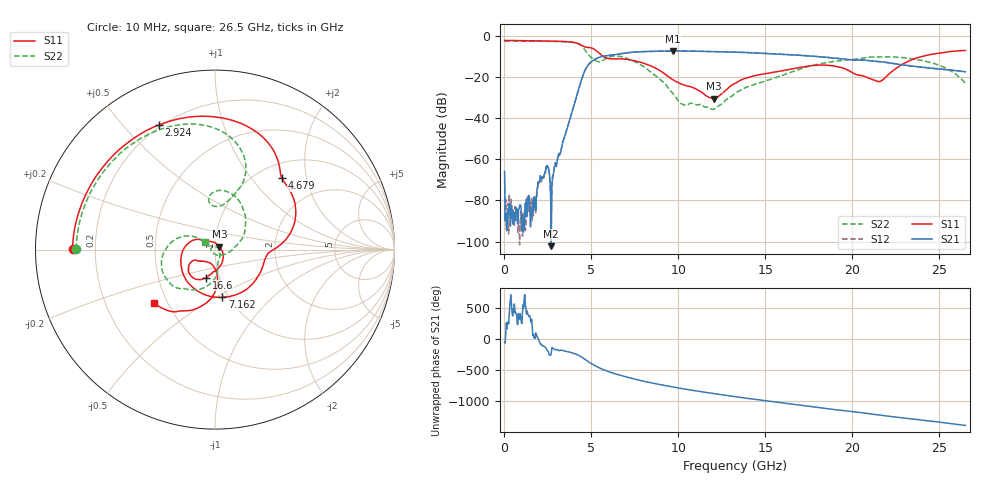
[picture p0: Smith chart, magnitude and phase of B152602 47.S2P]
!  2-Port S-parameters saved by WinCal
! VAR MeasName=S-Parameters (CALIBRATED_DATA) read from VNA (N5242A)
! VAR MeasDate=2016-1-5 16:32:53
! VAR NAME=B152602 47
! VAR FILENAME=B152602 47.S2P
! VAR DATE=2016-1-5 16:32:53
! VAR PHYS_PORTS=1,2
# Hz S DB R 50
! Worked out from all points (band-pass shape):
!   801 points, 10 MHz to 26.5 GHz, reference 50 ohm
!   highest |S21| = -7.09 dB at 9.679 GHz (marker M1); lowest = -102.3 dB at 2.692 GHz (marker M2)
!   |S21| within 3 dB of the highest: 5.494 GHz to 18.3 GHz (12.81 GHz wide, 108 % of centre)
!   lowest |S11| = -30.4 dB at 12.06 GHz (marker M3), VSWR 1.06, Z = 52.5 + j1.81 ohm
!   |S11| at or under -10 dB: 5.717 GHz to 23.92 GHz (18.2 GHz wide, 123 % of centre)
!   |S22| runs from -35.6 to -2.2 dB; largest |S21 - S12| = 0.0027
!   S11 on the Smith chart (normalised r, x): 10 MHz: 0.12, +0.00; 2.924 GHz: 0.19, +0.63; 4.679 GHz: 1.26, +1.44; 7.162 GHz: 0.93, -0.54; 16.6 GHz: 0.87, -0.28; 26.5 GHz: 0.42, -0.32
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1e7  -2.02 179.7  -65.84 -55.3  -70.16 -142.2  -2.24 179.8
1.755625e8  -2.02 176.4  -88.71 -84.1  -84.82 -162.3  -2.24 177.3
1.102712e9  -2.13 157.4  -94.88 143.0  -92.38 172.0  -2.30 162.9
1.73185e9  -2.20 143.9  -82.57 36.9  -82.17 30.6  -2.36 152.8
2.427212e9  -2.29 127.6  -64.22 -163.1  -64.13 -160.9  -2.44 140.5
2.692112e9  -2.32 120.7  -102.26 135.2  -88.88 -154.1  -2.46 135.4
2.9239e9  -2.36 114.2  -61.79 -168.0  -61.53 -163.7  -2.50 130.5
4.447075e9  -4.40 54.1  -20.74 69.9  -20.74 70.1  -4.73 76.0
4.678862e9  -5.26 47.1  -15.77 25.3  -15.79 25.4  -7.31 67.5
5.506675e9  -8.66 4.6  -10.05 -109.1  -10.06 -109.0  -12.31 91.4
6.23515e9  -10.98 -17.2  -9.05 173.0  -9.05 173.2  -9.68 87.7
7.1623e9  -11.40 -81.4  -7.92 99.2  -7.90 99.2  -11.16 55.5
8.851038e9  -16.27 167.1  -7.23 -7.3  -7.23 -7.4  -20.19 0.3
9.67885e9  -21.06 143.4  -7.09 -50.8  -7.10 -50.8  -27.80 -49.8
1.206295e10  -30.42 34.9  -7.44 -158.3  -7.46 -158.3  -35.35 51.5
1.3255e10  -22.92 -52.2  -7.73 153.8  -7.72 153.8  -27.87 -48.7
1.48444e10  -18.40 -91.0  -8.28 93.2  -8.24 93.1  -22.25 -77.8
1.659936e10  -15.76 -107.4  -9.08 29.2  -9.03 29.2  -17.10 -86.5
1.769208e10  -14.24 -121.0  -9.67 -9.8  -9.64 -9.6  -14.26 -98.2
2.209604e10  -18.45 -87.0  -12.93 -162.2  -12.88 -162.3  -9.98 -156.7
2.474504e10  -8.51 -114.8  -15.73 111.0  -15.68 110.8  -13.33 162.5
2.65e10  -6.87 -138.8  -17.31 49.2  -17.28 48.8  -22.95 144.2
